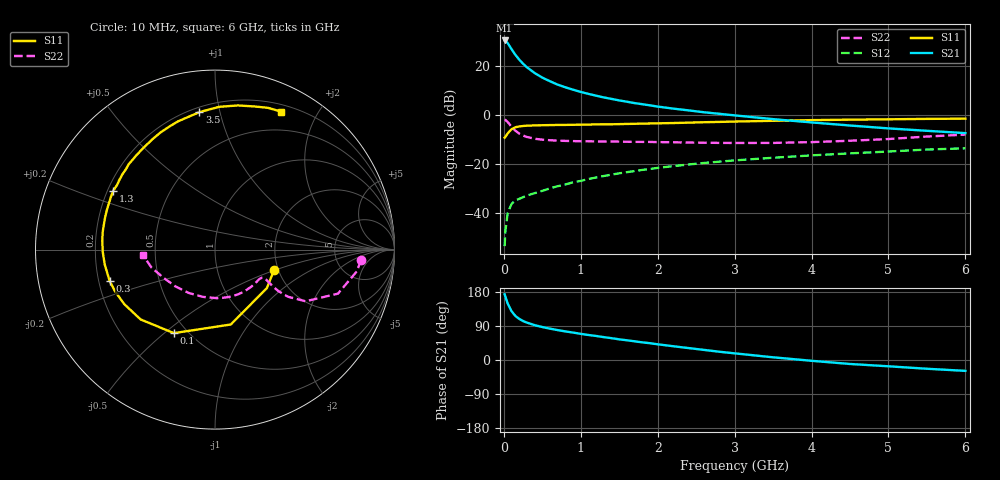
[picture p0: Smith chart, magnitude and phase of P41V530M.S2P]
! SIEMENS Small Signal Semiconductors
! BFP182
! Si NPN RF Bipolar Junction Transistor in SOT143
! VCE = 1.5 V  IC = 30 mA
! Common Emitter S-Parameters:  March  1996
# GHz  S  MA  R  50
!  f  S11  S21  S12  S22
! GHz  MAG  ANG  MAG  ANG  MAG  ANG  MAG  ANG
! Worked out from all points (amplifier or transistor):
!   36 points, 10 MHz to 6 GHz, reference 50 ohm
!   highest |S21| = 30.6 dB at 10 MHz (marker M1)
!   |S21| within 3 dB of that: start of sweep to 88.86 MHz
!   unconditionally stable (mu >= 1): start of sweep to 22.38 MHz; 234.6 MHz to end of sweep
!   at 250 MHz: K = 1.04, MAG = 26.1 dB, |S12| = -33.5 dB
!   at 1.4 GHz: K = 1.87, MAG = 10.1 dB, |S12| = -24.3 dB
!   at 6 GHz: K = 1.35, MAG = -0.4 dB, |S12| = -13.5 dB
!   S11 on the Smith chart (normalised r, x): 10 MHz: 1.90, -0.49; 100 MHz: 0.42, -0.54; 300 MHz: 0.25, -0.14; 1.3 GHz: 0.22, +0.26; 3.5 GHz: 0.23, +0.87; 6 GHz: 0.28, +1.56
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0.01  0.3482 -18.8  33.9 173.4  0.0021 80.2  0.8145 -4.0
0.02  0.3599 -36.5  33.52 167.1  0.0043 74.0  0.8013 -8.5
0.05  0.4264 -78.1  29.98 149.1  0.01 65.2  0.7277 -19.7
0.1  0.5186 -116.2  22.52 128.9  0.0153 51.2  0.5811 -29.7
0.15  0.5685 -136.8  17.25 116.4  0.0182 45.5  0.483 -32.9
0.2  0.5899 -149.0  13.76 108.5  0.0195 43.9  0.4212 -33.2
0.25  0.6033 -157.3  11.32 102.8  0.0211 44.6  0.3845 -32.5
0.3  0.6124 -163.4  9.58 98.6  0.0228 45.0  0.3598 -31.6
0.4  0.6199 -172.3  7.314 91.9  0.0255 48.4  0.3309 -30.4
0.5  0.6254 -178.7  5.894 87.0  0.0284 49.5  0.3166 -30.1
0.6  0.6297 175.8  4.963 82.7  0.032 51.8  0.3086 -30.5
0.7  0.6334 171.1  4.231 78.9  0.0354 53.6  0.3029 -31.3
0.8  0.6349 167.1  3.731 75.4  0.0384 55.1  0.2991 -32.6
1.1  0.6451 156.2  2.739 66.0  0.0497 56.6  0.2933 -37.6
1.3  0.6549 149.9  2.318 60.3  0.0573 56.7  0.2904 -41.6
1.7  0.6685 137.9  1.774 49.3  0.0722 55.2  0.2857 -50.5
2.2  0.6933 125.0  1.37 36.4  0.091 51.7  0.2802 -63.4
2.8  0.7313 110.3  1.072 21.8  0.1124 46.3  0.2722 -80.9
3.5  0.7706 96.5  0.833 7.1  0.1352 39.7  0.2718 -104.3
4.5  0.8132 81.0  0.617 -10.5  0.1662 30.3  0.3011 -137.1
5.5  0.8433 69.5  0.481 -23.1  0.199 20.7  0.3671 -164.0
6  0.8525 64.3  0.431 -28.7  0.2111 15.1  0.4026 -175.6
